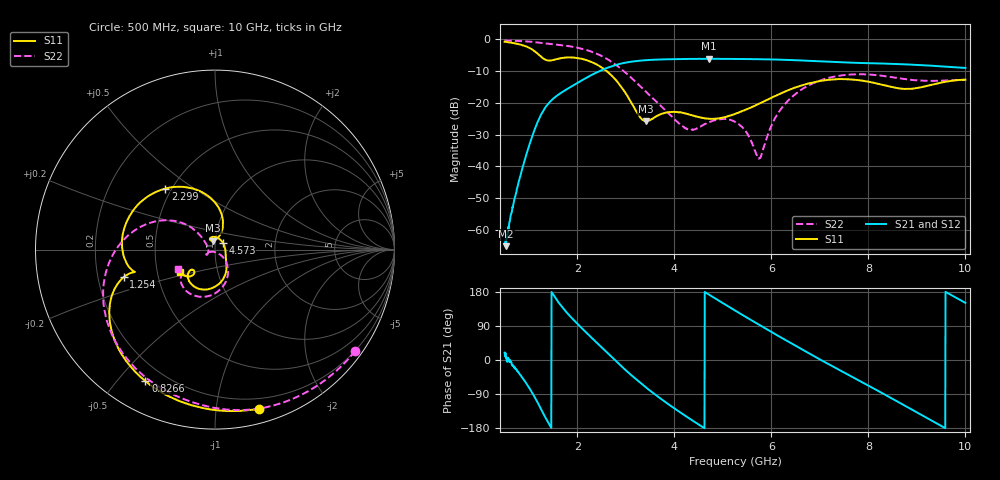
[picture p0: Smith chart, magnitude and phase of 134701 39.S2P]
!  2-Port S-parameters saved by WinCal
! VAR MeasName=S-Parameters (CALIBRATED_DATA) read from VNA (N5242A)
! VAR MeasDate=2013-7-3 16:37:25
! VAR NAME=134701 39
! VAR FILENAME=134701 39.S2P
! VAR DATE=2013-7-3 16:37:25
! VAR PHYS_PORTS=1,2
# Hz S MA R 50
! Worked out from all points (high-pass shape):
!   1601 points, 500 MHz to 10 GHz, reference 50 ohm
!   highest |S21| = -6.12 dB at 4.716 GHz (marker M1); lowest = -65.2 dB at 529.7 MHz (marker M2)
!   |S21| within 3 dB of the highest: 2.587 GHz to end of sweep
!   lowest |S11| = -25.9 dB at 3.415 GHz (marker M3), VSWR 1.11, Z = 48.8 + j4.88 ohm
!   |S11| at or under -10 dB: 2.605 GHz to end of sweep
!   |S22| runs from -37.6 to -0.3 dB; largest |S21 - S12| = 0.0019
!   S11 on the Smith chart (normalised r, x): 500 MHz: 0.11, -1.31; 826.6 MHz: 0.13, -0.59; 1.254 GHz: 0.31, -0.13; 2.299 GHz: 0.46, +0.39; 4.573 GHz: 1.09, +0.09; 10 GHz: 0.65, -0.17
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5e8  0.9203 -74.6  0.0006042 19.4  0.0006809 17.7  0.9629 -35.9
5.296875e8  0.9131 -78.7  0.0005512 8.4  0.0007001 9.9  0.9615 -38.0
8.265625e8  0.8289 -117.9  0.00716 -40.0  0.007193 -40.1  0.9419 -59.1
1.034375e9  0.7199 -144.1  0.02481 -79.4  0.0248 -79.4  0.9198 -73.9
1.254062e9  0.5305 -163.2  0.06569 -130.4  0.06564 -130.7  0.8835 -89.5
1.634062e9  0.5018 -172.4  0.1389 148.0  0.1386 147.8  0.8183 -115.2
2.085312e9  0.4958 149.2  0.2247 84.7  0.2238 84.7  0.7149 -148.2
2.299062e9  0.4381 129.1  0.2767 58.1  0.2753 58.1  0.6385 -164.9
2.869062e9  0.1946 78.6  0.4102 -11.9  0.4099 -11.8  0.3601 153.8
3.415312e9  0.05088 101.3  0.4701 -72.4  0.47 -72.4  0.1495 135.9
3.670625e9  0.0636 116.6  0.482 -97.6  0.4811 -97.5  0.09768 137.6
4.246562e9  0.06755 78.5  0.4926 -149.1  0.4921 -149.0  0.03943 173.4
4.573125e9  0.05812 42.2  0.4938 -176.1  0.4937 -176.1  0.04401 -153.2
4.715625e9  0.0561 24.5  0.4944 172.4  0.4942 172.4  0.04963 -147.9
5.25e9  0.06697 -27.5  0.4919 130.6  0.4923 130.6  0.0502 -154.1
5.754688e9  0.09758 -49.6  0.4873 92.4  0.4876 92.4  0.01347 -97.0
6.188125e9  0.14 -64.2  0.4791 60.2  0.4799 60.2  0.07815 -45.7
6.835312e9  0.2076 -90.6  0.4581 13.2  0.4588 13.2  0.2003 -74.8
7.714062e9  0.2315 -126.2  0.4288 -47.9  0.4287 -48.1  0.2813 -115.2
8.420625e9  0.1825 -140.2  0.4142 -97.2  0.4128 -97.2  0.2587 -137.7
9.24e9  0.1876 -130.9  0.3873 -155.3  0.3876 -155.3  0.2218 -144.7
1e10  0.2321 -147.9  0.3558 150.7  0.3558 150.6  0.2295 -152.5
